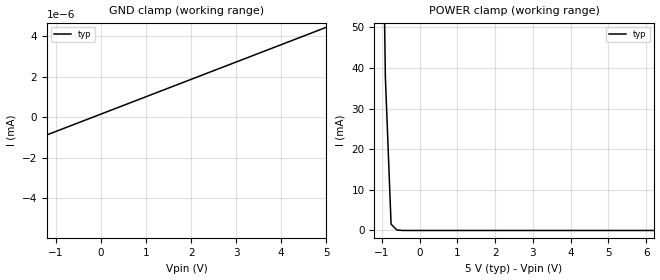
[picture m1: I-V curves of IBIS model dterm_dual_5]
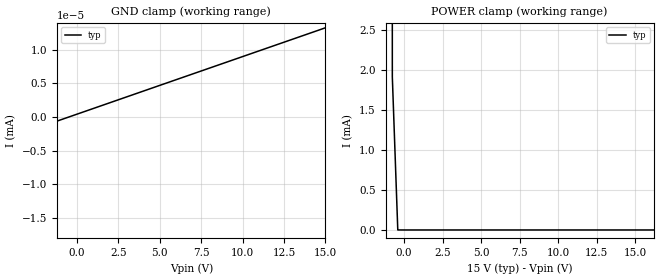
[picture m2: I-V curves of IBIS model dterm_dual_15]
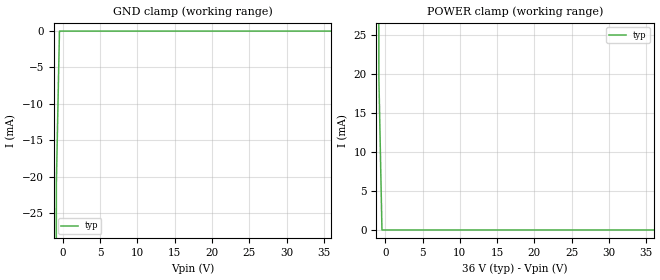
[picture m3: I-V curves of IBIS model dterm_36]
|Texas Instruments Incorporated
|tmux6236, 2 Data Lane 2:1 36V Precision mux
[IBIS Ver]   4.1
[File name]   tmux6236.ibs
[Date]   04/13/22
[File Rev]   1.0
[Source]
| Texas Instruments Incorporated.
| ASC-INT-MPD
| 12500 TI Blvd
| Dallas, TX - 75243
[Notes]   Revision History:
| Rev 1.0: 04/13/22
| - Initial version of the model
| - Model generated from simulations in SPECTRE
| - C_comp although listed in numerical order of value are
|   obtained from varying PVT conditions. For PVT conditions for
|   each specific value refer the buffer description under
|   respective [Model]. IBIS model user is responsible for using
|   appropriate C_comp to simulate for Signal Integrity.
[Disclaimer]
| This model is designed as an aid for customers of Texas Instruments.
| TI and its licensors and suppliers make no warranties, either expressed
| or implied, with respect to this  model, including the warranties of
| merchantability or fitness for a particular purpose. The model is
| provided solely on an "as is" basis. The entire risk as to its quality
| and performance is with the customer.
| This model is subject to change without notice. Texas Instruments
| Incorporated is not responsible for updating this model.
[Copyright]
(C) Copyright 2022 Texas Instruments Incorporated.All rights reserved.
|  Component TMUX6236PW 16-pin - PW package
|  Part # TMUX6236PW
[Component]   TMUX6236PW
[Manufacturer]  TI
[Package]
|   typ   min   max
R_pkg   0.05   NA   NA
L_pkg   1.0nH   NA   NA
C_pkg   0.2pF   NA   NA
[Pin]   signal_name   model_name
   1   SEL1   inbuf
   2   S1A   sterm
   3   D1   dterm
   4   S1B   sterm
   5   VSS   power
   6   GND   gnd
   7   NC   nc
   8   NC   nc
   9   SEL2   inbuf
   10   S2A   sterm
   11   D2   dterm
   12   S2B   sterm
   13   VDD   power
   14   EN   inbuf
   15   NC   nc
   16   NC   nc
[Series Switch Groups]
On 1 /
On 2 /
Off 1 2 /
[Series Pin Mapping]  pin_2 model_name function_table_group
|  2   3   switch_dual_5   1
|  10  11   switch_dual_5   1
|   4   3   switch_dual_5   2
|  12  11   switch_dual_5   2
   2   3   switch_dual_15   1
  10  11   switch_dual_15   1
   4   3   switch_dual_15   2
  12  11   switch_dual_15   2
|   2   3   switch_36   1
|  10  11   switch_36   1
|   4   3   switch_36   2
|  12  11   switch_36   2
|   2   3   switch_12   1
|  10  11   switch_12   1
|   4   3   switch_12   2
|  12  11   switch_12   2
|  Component TMUX6236RUM 16-pin - RUM package
|  Part # TMUX6236RUM
[Component]   TMUX6236RUM
[Manufacturer]  TI
[Package]
|   typ   min   max
R_pkg   0.05   NA   NA
L_pkg   1.0nH   NA   NA
C_pkg   0.2pF   NA   NA
[Pin]   signal_name   model_name
   1   D1   dterm
   2   S1B   sterm
   3   VSS   power
   4   GND   gnd
   5   NC   nc
   6   SEL2   inbuf
   7   NC   nc
   8   S2A   sterm
   9   D2   dterm
   10   S2B   sterm
   11   VDD   power
   12   EN   inbuf
   13   NC   nc
   14   NC   nc
   15   SEL1   inbuf
   16   S1A   sterm
[Series Switch Groups]
On 1 /
On 2 /
Off 1 2 /
[Series Pin Mapping]  pin_2 model_name function_table_group
|  16   1   switch_dual_5   1
|   8   9   switch_dual_5   1
|   2   1   switch_dual_5   2
|  10   9   switch_dual_5   2
  16   1   switch_dual_15   1
   8   9   switch_dual_15   1
   2   1   switch_dual_15   2
  10   9   switch_dual_15   2
|  16   1   switch_36   1
|   8   9   switch_36   1
|   2   1   switch_36   2
|  10   9   switch_36   2
|  16   1   switch_12   1
|   8   9   switch_12   1
|   2   1   switch_12   2
|  10   9   switch_12   2
[Model Selector] dterm
dterm_dual_5 Use for operation at +/-5V
dterm_dual_15 Use for operation at +/-15V
dterm_36 Use for operation at 36V
dterm_12 Use for operation at 12V
[Model Selector] sterm
sterm_dual_5 Use for operation at +/-5V
sterm_dual_15 Use for operation at +/-15V
sterm_36 Use for operation at 36V
sterm_12 Use for operation at 12V
[Model Selector] inbuf
inbuf_dual_5 Use for operation at +/-5V
inbuf_dual_15 Use for operation at +/-15V
inbuf_36 Use for operation at 36V
inbuf_12 Use for operation at 12V
| switch_dual_5
[Model]   switch_dual_5
Model_type   Series_switch
|   typ   min   max
C_comp   2.533030e-11   NA   NA
[Voltage Range]   5   NA   NA
[Power Clamp Reference]   5   NA   NA
[Temperature Range]   27   NA   NA
[On]
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[Off]
|   typ   min   max
[R Series]   10G   NA   NA
| switch_dual_15
[Model]   switch_dual_15
Model_type   Series_switch
|   typ   min   max
C_comp   4.014581e-11   NA   NA
[Voltage Range]   15   NA   NA
[Power Clamp Reference]   15   NA   NA
[Temperature Range]   27   NA   NA
[On]
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[Off]
|   typ   min   max
[R Series]   10G   NA   NA
| switch_36
[Model]   switch_36
Model_type   Series_switch
|   typ   min   max
C_comp   2.533030e-11   NA   NA
[Voltage Range]   36   NA   NA
[Power Clamp Reference]   36   NA   NA
[Temperature Range]   27   NA   NA
[On]
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[Off]
|   typ   min   max
[R Series]   10G   NA   NA
| switch_12
[Model]   switch_12
Model_type   Series_switch
|   typ   min   max
C_comp   2.533030e-11   NA   NA
[Voltage Range]   12   NA   NA
[Power Clamp Reference]   12   NA   NA
[Temperature Range]   27   NA   NA
[On]
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[Off]
|   typ   min   max
[R Series]   10G   NA   NA
| Models and submodels in the file (16): dterm_dual_5 (Terminator), dterm_dual_15 (Terminator), dterm_36 (Terminator), dterm_12 (Terminator), switch_dual_5 (Series_switch), switch_dual_15 (Series_switch), switch_36 (Series_switch), switch_12 (Series_switch), sterm_dual_5 (Terminator), sterm_dual_15 (Terminator), sterm_36 (Terminator), sterm_12 (Terminator), inbuf_dual_5 (Input), inbuf_dual_15 (Input), inbuf_36 (Input), inbuf_12 (Input)
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| dterm_dual_5
[Model]   dterm_dual_5
Model_type   Terminator
|   typ   min   max
C_comp   2.533030e-11   NA   NA
[Voltage Range]   5   NA   NA
[Temperature Range]   27   NA   NA
[Power Clamp Reference]   5   NA   NA
[GND Clamp Reference]   0   NA   NA
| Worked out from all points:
|   GND clamp passes 1 mA (typ) near -5.68 V on its own axis
|   POWER clamp passes 1 mA (typ) near -0.70 V on its own axis
[GND Clamp]
|   Voltage   I(typ)   I(min)   I(max)
-10V      -7.788A    NA         NA
-5.303V   -22.09nA   NA         NA
-5.152V   -5.127nA   NA         NA
-5V       -4.133nA   NA         NA
5V        4.429nA    NA         NA
[POWER Clamp]
|   Voltage   I(typ)   I(min)   I(max)
-5V       10.12A     NA         NA
-1.061V   139.4mA    NA         NA
-909.1mV  37.82mA    NA         NA
-757.6mV  1.557mA    NA         NA
-606.1mV  127.8uA    NA         NA
10V       -4.133nA   NA         NA
| dterm_dual_15
[Model]   dterm_dual_15
Model_type   Terminator
|   typ   min   max
C_comp   4.014581e-11   NA   NA
[Voltage Range]   15   NA   NA
[Temperature Range]   27   NA   NA
[Power Clamp Reference]   15   NA   NA
[GND Clamp Reference]   0   NA   NA
[GND Clamp]
|   Voltage   I(typ)   I(min)   I(max)
-20V      -8.063A    NA         NA
-15.4V    -362.8nA   NA         NA
-15.05V   -12.47nA   NA         NA
15V       13.28nA    NA         NA
[POWER Clamp]
|   Voltage   I(typ)   I(min)   I(max)
-5V       10.14A     NA         NA
-1.111V   212mA      NA         NA
-757.6mV  1.912mA    NA         NA
-404mV    417.9nA    NA         NA
30V       -12.41nA   NA         NA
| dterm_36
[Model]   dterm_36
Model_type   Terminator
|   typ   min   max
C_comp   4.014581e-11   NA   NA
[Voltage Range]   36   NA   NA
[Temperature Range]   27   NA   NA
[Power Clamp Reference]   36   NA   NA
[GND Clamp Reference]   0   NA   NA
[GND Clamp]
|   Voltage   I(typ)   I(min)   I(max)
-5V       -8.114A    NA         NA
-1.273V   -450.1mA   NA         NA
-858.6mV  -21.02mA   NA         NA
-444.4mV  -1.252uA   NA         NA
36V       15.94nA    NA         NA
[POWER Clamp]
|   Voltage   I(typ)   I(min)   I(max)
-5V       10.15A     NA         NA
-1.273V   460mA      NA         NA
-858.6mV  19.58mA    NA         NA
-444.4mV  1.492uA    NA         NA
36V       -14.91nA   NA         NA
